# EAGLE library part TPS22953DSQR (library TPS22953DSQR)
5.7V, 5A, 14m Load Switch with Voltage Monitoring and Reverse Current Protection Source: Datasheet
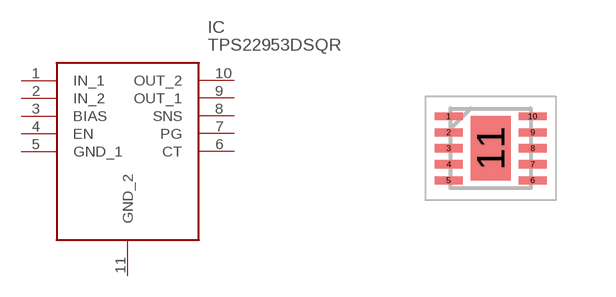
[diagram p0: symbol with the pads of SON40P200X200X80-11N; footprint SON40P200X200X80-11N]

Designator prefix IC

## TPS22953DSQR (Description: 5.7V, 5A, 14m Load Switch with Voltage Monitoring and Reverse Current Protection; Height: 0.8mm; Manufacturer_Name: Texas Instruments; Manufacturer_Part_Number: TPS22953DSQR; Mouser_Part_Number: 595-TPS22953DSQR; Mouser_Price-Stock: https://www.mouser.co.uk/ProductDetail/Texas-Instruments/TPS22953DSQR?qs=lGsJEpdjMw3By0yQoF%252B7vQ%3D%3D)  [SON40P200X200X80-11N]
1  IN_1
2  IN_2
3  BIAS
4  EN
5  GND_1
6  CT
7  PG
8  SNS
9  OUT_1
10  OUT_2
11  GND_2

## Footprint SON40P200X200X80-11N (pad centres in mm)
DSQ0010A
smd 0.7 x 0.2: 1 -1.05,0.8; 2 -1.05,0.4; 3 -1.05,0; 4 -1.05,-0.4; 5 -1.05,-0.8; 6 1.05,-0.8; 7 1.05,-0.4; 8 1.05,0; 9 1.05,0.4; 10 1.05,0.8
smd 1 x 1.6: 11 0,0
